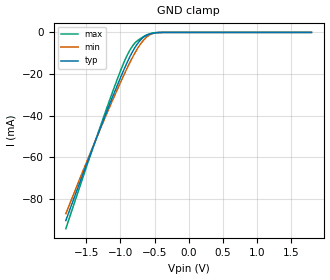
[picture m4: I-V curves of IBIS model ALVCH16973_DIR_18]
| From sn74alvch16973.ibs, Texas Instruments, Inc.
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[Model]   ALVCH16973_DIR_18
Model_type  Input
Vinl=0.5775
Vinh=1.2675
| variable   typ   min   max
C_comp   2.61pF   2.20pF   3.10pF
[Temperature Range]   40   100   -40
| Ambient temperature   25   85   -40
[Voltage range]   1.8   1.65   1.95
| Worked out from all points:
|   GND clamp passes 1 mA (typ) near -0.58 V on its own axis
[GND Clamp]
| ALVCH16973_DIR_18
|   Voltage   I(typ)   I(min)   I(max)
-1.8V     -90.36mA   -87.06mA   -94.23mA
-1.34V    -49.88mA   -49.94mA   -49.51mA
-1.03V    -24.19mA   -26.29mA   -21.12mA
-945mV    -17.65mA   -20.18mA   -14.16mA
-880mV    -12.98mA   -15.72mA   -9.673mA
-815mV    -8.831mA   -11.53mA   -6.213mA
-750mV    -5.474mA   -7.789mA   -3.976mA
-675mV    -2.681mA   -4.31mA    -2.304mA
-600mV    -1.199mA   -1.844mA   -1.035mA
-535mV    -533.8uA   -655.1uA   -350.4uA
-455mV    -127.2uA   -144.7uA   -47.79uA
1.8V      127.8pA    817.9pA    24.46pA
